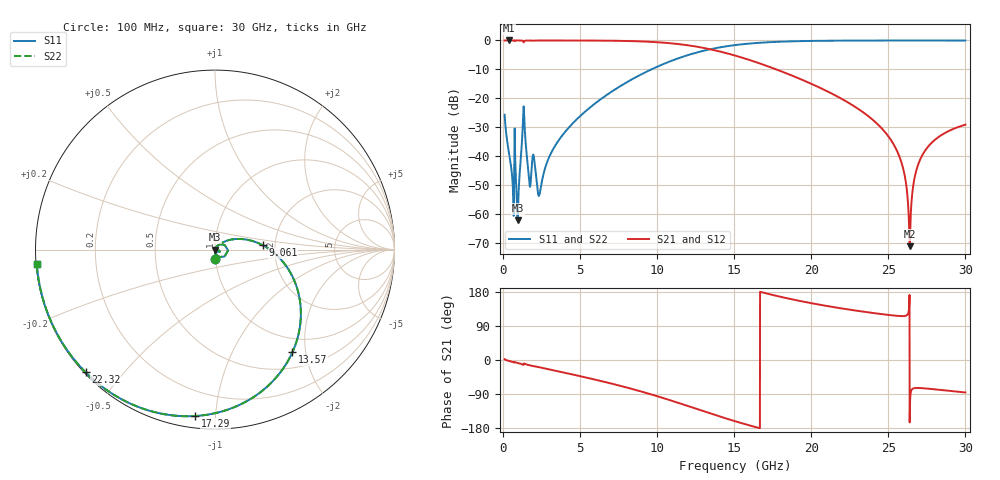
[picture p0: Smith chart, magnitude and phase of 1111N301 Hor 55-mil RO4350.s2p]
# GHz S MA R 50
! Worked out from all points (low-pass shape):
!   3201 points, 100 MHz to 30 GHz, reference 50 ohm
!   highest |S21| = 0.00 dB at 371 MHz (marker M1); lowest = -71.1 dB at 26.38 GHz (marker M2)
!   |S21| within 3 dB of the highest: start of sweep to 13.4 GHz
!   lowest |S11| = -62.2 dB at 940.9 MHz (marker M3), VSWR 1.00, Z = 50.1 - j0.0052 ohm
!   |S11| at or under -10 dB: start of sweep to 9.624 GHz
!   |S22| runs from -62.2 to 0.0 dB; largest |S21 - S12| = 5.6e-11
!   S11 on the Smith chart (normalised r, x): 100 MHz: 1.00, -0.10; 9.061 GHz: 1.72, +0.09; 13.57 GHz: 0.75, -1.76; 17.29 GHz: 0.06, -0.89; 22.32 GHz: 0.00, -0.40; 30 GHz: 0.00, -0.04
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0.1  0.05217 -87.6  0.9984 2.2  0.9984 2.2  0.05217 -87.6
0.3709688  0.01199 -90.5  0.9995 -2.4  0.9995 -2.4  0.01199 -90.5
0.9409375  0.0007793 -3.8  0.9991 -7.7  0.9991 -7.7  0.0007793 -3.8
1.333375  0.07311 -3.7  0.9274 -11.5  0.9274 -11.5  0.07311 -3.7
1.679094  0.004115 -68.4  0.9974 -13.5  0.9974 -13.5  0.004115 -68.4
1.996781  0.009794 -40.4  0.9908 -16.0  0.9908 -16.0  0.009794 -40.4
2.351844  0.002121 6.5  0.9978 -19.2  0.9978 -19.2  0.002121 6.5
3.248844  0.01324 57.5  0.9983 -27.0  0.9983 -27.0  0.01324 57.5
5.089563  0.05184 45.0  0.9967 -43.4  0.9967 -43.4  0.05184 45.0
9.060656  0.2671 5.2  0.9602 -84.2  0.9602 -84.2  0.2671 5.2
10.06978  0.3582 -6.8  0.9298 -96.4  0.9298 -96.4  0.3582 -6.8
13.57369  0.7164 -53.0  0.6917 -142.6  0.6917 -142.6  0.7164 -53.0
15.05  0.8313 -71.8  0.5486 -161.5  0.5486 -161.5  0.8313 -71.8
17.2925  0.9335 -96.7  0.3489 173.6  0.3489 173.6  0.9335 -96.7
20.03956  0.9814 -120.7  0.1764 149.6  0.1764 149.6  0.9814 -120.7
22.31944  0.9935 -136.5  0.08681 133.9  0.08681 133.9  0.9935 -136.5
25.01978  0.9971 -152.1  0.02173 118.8  0.02173 118.8  0.9971 -152.1
25.91678  0.9973 -156.8  0.006804 115.8  0.006804 115.8  0.9973 -156.8
26.38397  0.9974 -159.1  0.0002794 -164.6  0.0002794 -164.6  0.9974 -159.1
26.76706  0.9973 -161.0  0.005071 -73.9  0.005071 -73.9  0.9973 -161.0
27.309  0.9973 -163.6  0.01162 -74.7  0.01162 -74.7  0.9973 -163.6
30  0.9966 -175.5  0.03511 -85.7  0.03511 -85.7  0.9966 -175.5
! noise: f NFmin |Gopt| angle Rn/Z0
0.1  0.0006655  0.7343  0.9638  0.0005002
3.417  0.009296  0.4634  27.31  0.002778
6.743  0.01543  0.4142  49.89  0.003658
10.06  0.02381  0.4584  68.07  0.005389
13.39  0.03745  0.5635  85.16  0.008926
16.7  0.06457  0.7078  104.1  0.01724
20.03  0.1327  0.8462  124.3  0.041
23.35  0.3904  0.9447  143.5  0.1564
26.67  5.533  0.9953  160.5  10.11
30  0.6796  0.9653  175.5  0.008368
